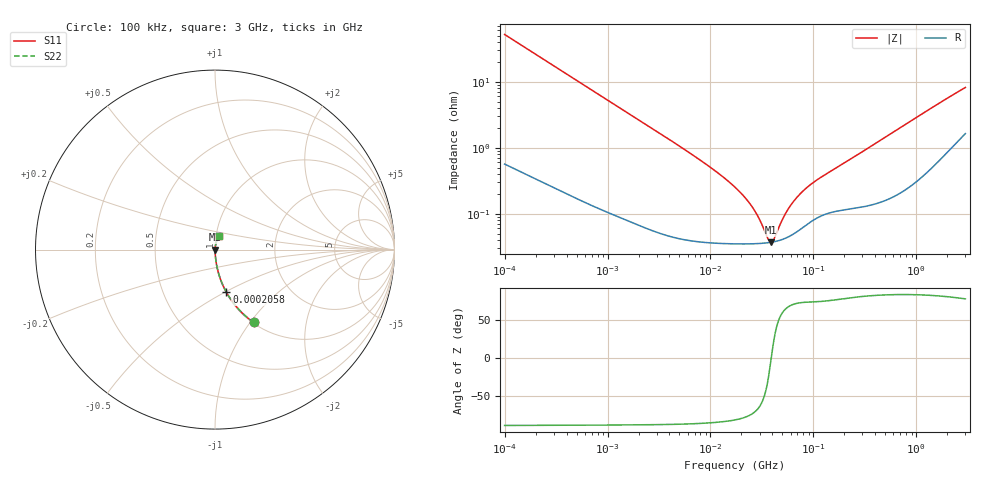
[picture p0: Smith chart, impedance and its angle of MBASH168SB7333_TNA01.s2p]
! MBASH168SB7333_TNA01  S-PARAMETER MODEL  ( Standard Model )
! Model Generated by TAIYO YUDEN Corporation (http://www.ty-top.com)
! Version 1.0
! TAIYO YUDEN Control No. 220601
! Copyright(c) 2013 TAIYO YUDEN CO.,LTD. All Rights Reserved.
! Product Description (link to TY-COMPAS)
! https://ds.yuden.co.jp/TYCOMPAS/or/detail?pn=MBASH168SB7333KTNA01&u=M
! Products Name : Multilayer Ceramic Capacitors
! Characteristics :
!  Capacitance : 0.033 [uF] , Rated Voltage : 100 [V] , TCC : X7R
!  Case Size : 1.6 x 0.8 / 0.063 x 0.031 [mm/inch] , Thickness : 0.8 / 0.031 [mm/inch]
!  (Conditions: Temperature = 25 [degC] , DC Bias Voltage = 0 [V])
! External Node Assignments :
!  1  o---| |---o  2
! GND o---------o GND
! Frequency Range : 100kHz  -  3GHz  [ 401 STEP ]
# MHZ S RI R 50
! Freq[MHz].  S11 Real  S11 Imag  S21 Real  S21 Imag  S12 Real  S12 Imag  S22 Real  S22 Imag
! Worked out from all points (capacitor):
!   401 points, 100 kHz to 3 GHz, reference 50 ohm
!   read as one part in series: C = 30.6 nF near 105.3 kHz
!   lowest |Z| = 37.1 mohm at 38.51 MHz (marker M1)
!   series resonance near 38.98 MHz, so ESL is about 550 pH
!   S11 on the Smith chart (normalised r, x): 100 kHz: 1.01, -1.04; 205.8 kHz: 1.01, -0.51; 3 GHz: 1.03, +0.16
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0.1  0.2151 -0.4055  0.7849 0.4055  0.7849 0.4055  0.2151 -0.4055
0.14345  0.1194 -0.3184  0.8806 0.3184  0.8806 0.3184  0.1194 -0.3184
0.205778  0.0632 -0.237  0.9368 0.237  0.9368 0.237  0.0632 -0.237
0.335785  0.0259 -0.1518  0.9741 0.1518  0.9741 0.1518  0.0259 -0.1518
0.562235  0.0102 -0.0926  0.9898 0.0926  0.9898 0.0926  0.0102 -0.0926
1.18716  0.00292 -0.0445  0.9971 0.0445  0.9971 0.0445  0.00292 -0.0445
3.161081  0.000794 -0.0168  0.9992 0.0168  0.9992 0.0168  0.000794 -0.0168
9.574722  0.000392 -0.00528  0.9996 0.00528  0.9996 0.00528  0.000392 -0.00528
17.7727  0.000356 -0.00241  0.9996 0.00241  0.9996 0.00241  0.000356 -0.00241
21.84217  0.000352 -0.0017  0.9996 0.0017  0.9996 0.0017  0.000352 -0.0017
26.16047  0.000353 -0.00114  0.9996 0.00114  0.9996 0.00114  0.000353 -0.00114
29.75839  0.000355 -0.000762  0.9996 0.000762  0.9996 0.000762  0.000355 -0.000762
35.64176  0.000363 -0.00025  0.9996 0.00025  0.9996 0.00025  0.000363 -0.00025
38.50681  0.000369 -3.37e-05  0.9996 3.37e-05  0.9996 3.37e-05  0.000369 -3.37e-05
41.60216  0.000378 0.000183  0.9996 -0.000183  0.9996 -0.000183  0.000378 0.000183
51.12795  0.000415 0.000773  0.9996 -0.000773  0.9996 -0.000773  0.000415 0.000773
61.23616  0.000475 0.00131  0.9995 -0.00131  0.9995 -0.00131  0.000475 0.00131
75.25761  0.000589 0.00195  0.9994 -0.00195  0.9994 -0.00195  0.000589 0.00195
97.38194  0.000787 0.00278  0.9992 -0.00278  0.9992 -0.00278  0.000787 0.00278
547.5153  0.00193 0.0157  0.9981 -0.0157  0.9981 -0.0157  0.00193 0.0157
1701.687  0.00875 0.047  0.9912 -0.047  0.9912 -0.047  0.00875 0.047
3000  0.0222 0.0771  0.9778 -0.0771  0.9778 -0.0771  0.0222 0.0771
